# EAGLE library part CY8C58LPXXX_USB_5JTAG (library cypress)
CY8C58LPXXX_TQFP100_USB_5JTAG edit this description Auto generated by make-symbol-device-package-bsdl.ulp Rev. 43 Source: CY8C58LPXXX_TQFP100_USB_5JTAG.bsdl
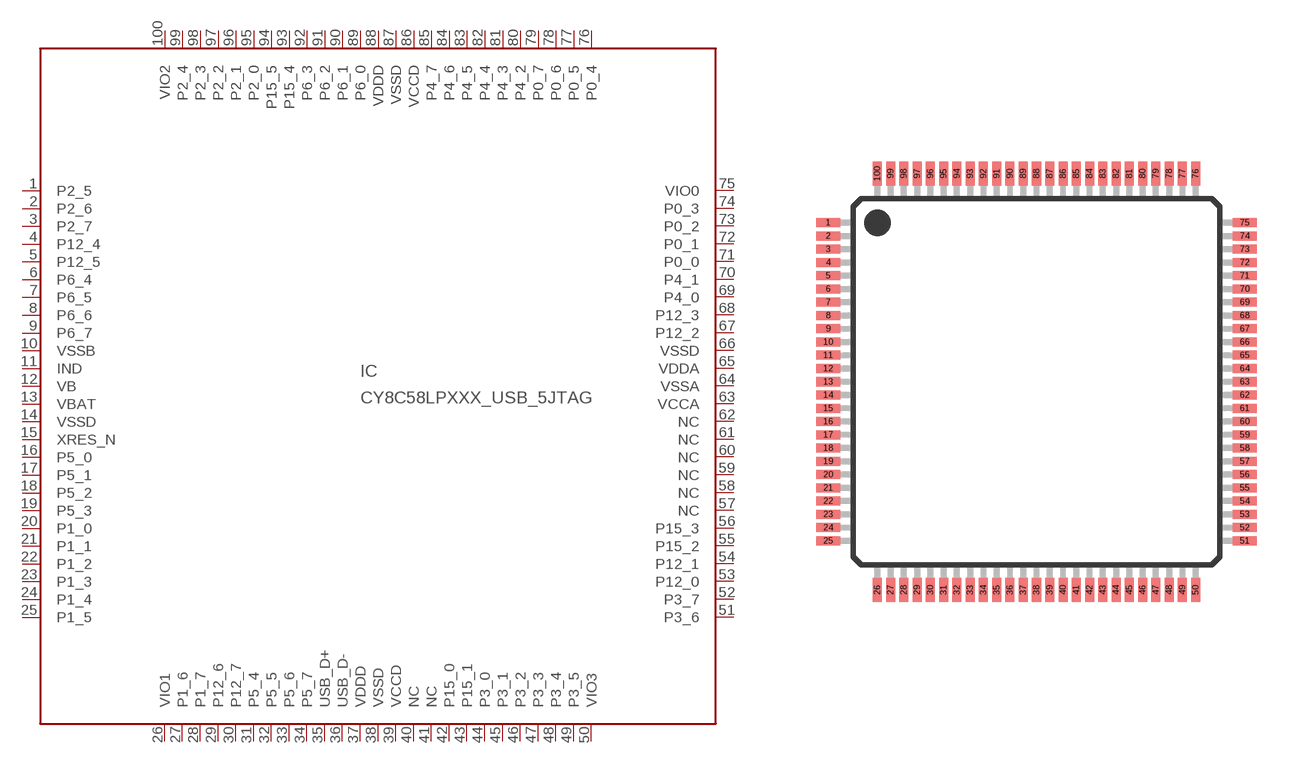
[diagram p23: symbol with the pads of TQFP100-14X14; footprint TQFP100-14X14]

Designator prefix IC

## CY8C58LPXXX_USB_5JTAG  [TQFP100-14X14]
1  P2_5
2  P2_6
3  P2_7
4  P12_4
5  P12_5
6  P6_4
7  P6_5
8  P6_6
9  P6_7
10  VSSB  pwr
11  IND  pas
12  VB  pas
13  VBAT  pas
14  VSSD  pwr
15  XRES_N  in
16  P5_0
17  P5_1
18  P5_2
19  P5_3
20  P1_0  in
21  P1_1  in
22  P1_2
23  P1_3  out
24  P1_4  in
25  P1_5  in
26  VIO1  pas
27  P1_6
28  P1_7
29  P12_6
30  P12_7
31  P5_4
32  P5_5
33  P5_6
34  P5_7
35  USB_D+  hiz
36  USB_D-  hiz
37  VDDD  pwr
38  VSSD  pwr
39  VCCD  pwr
40  NC  nc
41  NC  nc
42  P15_0
43  P15_1
44  P3_0
45  P3_1
46  P3_2
47  P3_3
48  P3_4
49  P3_5
50  VIO3  pas
51  P3_6
52  P3_7
53  P12_0
54  P12_1
55  P15_2
56  P15_3
57  NC  nc
58  NC  nc
59  NC  nc
60  NC  nc
61  NC  nc
62  NC  nc
63  VCCA  pwr
64  VSSA  pwr
65  VDDA  pwr
66  VSSD  pwr
67  P12_2
68  P12_3
69  P4_0
70  P4_1
71  P0_0
72  P0_1
73  P0_2
74  P0_3
75  VIO0  pas
76  P0_4
77  P0_5
78  P0_6
79  P0_7
80  P4_2
81  P4_3
82  P4_4
83  P4_5
84  P4_6
85  P4_7
86  VCCD  pwr
87  VSSD  pwr
88  VDDD  pwr
89  P6_0
90  P6_1
91  P6_2
92  P6_3
93  P15_4
94  P15_5
95  P2_0
96  P2_1
97  P2_2
98  P2_3
99  P2_4
100  VIO2  pas

## Footprint TQFP100-14X14 (pad centres in mm)
TQFP100 Auto generated by make-symbol-device-package-bsdl.ulp Rev. 43
smd 0.9 x 0.34: 1 -7.85,6; 2 -7.85,5.5; 3 -7.85,5; 4 -7.85,4.5; 5 -7.85,4; 6 -7.85,3.5; 7 -7.85,3; 8 -7.85,2.5; 9 -7.85,2; 10 -7.85,1.5; 11 -7.85,1; 12 -7.85,0.5; 13 -7.85,0; 14 -7.85,-0.5; 15 -7.85,-1; 16 -7.85,-1.5; 17 -7.85,-2; 18 -7.85,-2.5; 19 -7.85,-3; 20 -7.85,-3.5; 21 -7.85,-4; 22 -7.85,-4.5; 23 -7.85,-5; 24 -7.85,-5.5; 25 -7.85,-6; 51 7.85,-6; 52 7.85,-5.5; 53 7.85,-5; 54 7.85,-4.5; 55 7.85,-4; 56 7.85,-3.5; 57 7.85,-3; 58 7.85,-2.5; 59 7.85,-2; 60 7.85,-1.5; 61 7.85,-1; 62 7.85,-0.5; 63 7.85,0; 64 7.85,0.5; 65 7.85,1; 66 7.85,1.5; 67 7.85,2; 68 7.85,2.5; 69 7.85,3; 70 7.85,3.5; 71 7.85,4; 72 7.85,4.5; 73 7.85,5; 74 7.85,5.5; 75 7.85,6
smd 0.34 x 0.9: 26 -6,-7.85; 27 -5.5,-7.85; 28 -5,-7.85; 29 -4.5,-7.85; 30 -4,-7.85; 31 -3.5,-7.85; 32 -3,-7.85; 33 -2.5,-7.85; 34 -2,-7.85; 35 -1.5,-7.85; 36 -1,-7.85; 37 -0.5,-7.85; 38 0,-7.85; 39 0.5,-7.85; 40 1,-7.85; 41 1.5,-7.85; 42 2,-7.85; 43 2.5,-7.85; 44 3,-7.85; 45 3.5,-7.85; 46 4,-7.85; 47 4.5,-7.85; 48 5,-7.85; 49 5.5,-7.85; 50 6,-7.85; 76 6,7.85; 77 5.5,7.85; 78 5,7.85; 79 4.5,7.85; 80 4,7.85; 81 3.5,7.85; 82 3,7.85; 83 2.5,7.85; 84 2,7.85; 85 1.5,7.85; 86 1,7.85; 87 0.5,7.85; 88 0,7.85; 89 -0.5,7.85; 90 -1,7.85; 91 -1.5,7.85; 92 -2,7.85; 93 -2.5,7.85; 94 -3,7.85; 95 -3.5,7.85; 96 -4,7.85; 97 -4.5,7.85; 98 -5,7.85; 99 -5.5,7.85; 100 -6,7.85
